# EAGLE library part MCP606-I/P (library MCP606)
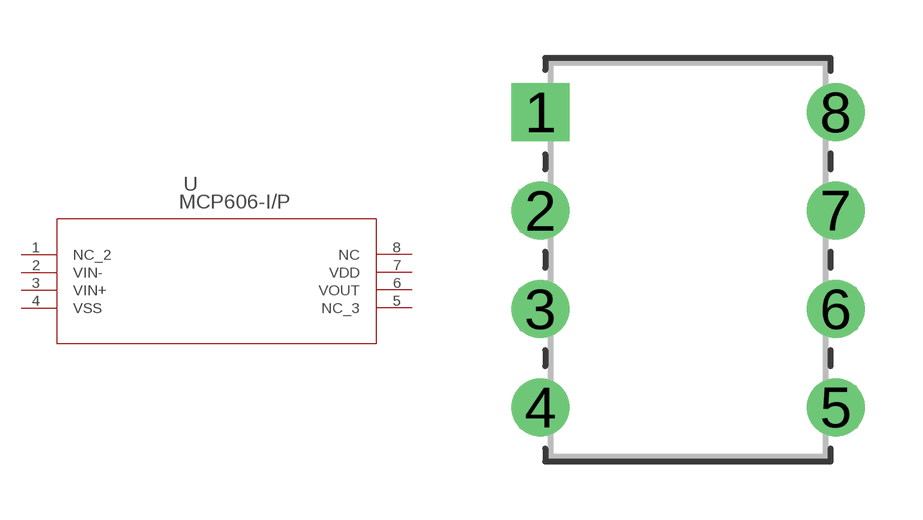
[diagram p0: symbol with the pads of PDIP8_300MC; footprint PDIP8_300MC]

Designator prefix U

## MCP606-I/P (MANUFACTURER_PART_NUMBER: MCP606IP; VENDOR: Microchip)  [PDIP8_300MC]
1  NC_2  pas
2  VIN-  pas
3  VIN+  pas
4  VSS  pas
5  NC_3  pas
6  VOUT  pas
7  VDD  pas
8  NC  pas

## Footprint PDIP8_300MC (pad centres in mm)
drill 0.991 pad 1.499 square: 1 -7.62,7.62
drill 0.991 pad 1.499: 2 -7.62,5.08; 3 -7.62,2.54; 4 -7.62,0; 5 0,0; 6 0,2.54; 7 0,5.08; 8 0,7.62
